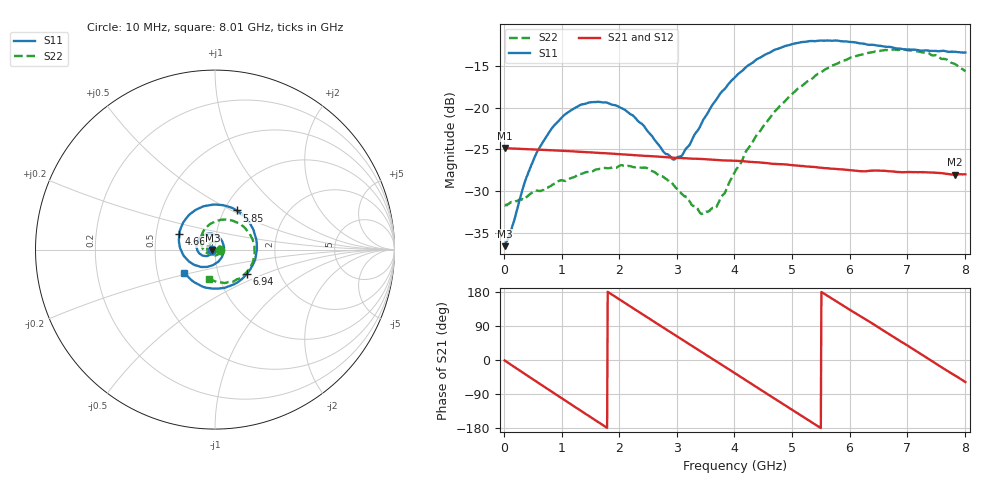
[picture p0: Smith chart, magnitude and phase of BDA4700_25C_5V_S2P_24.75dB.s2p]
!Agilent Technologies,E5071B,MY42404982,A.09.10
!Date: Mon Oct 20 13:38:55 2025
!Data & Calibration Information:
!Freq	S11:SOLT2(ON)	S21:SOLT2(ON)	S12:SOLT2(ON)	S22:SOLT2(ON)
# Hz S RI R 50
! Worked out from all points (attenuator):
!   801 points, 10 MHz to 8.01 GHz, reference 50 ohm
!   highest |S21| = -24.83 dB at 20 MHz (marker M1); lowest = -28.0 dB at 7.83 GHz (marker M2)
!   lowest |S11| = -36.6 dB at 10 MHz (marker M3), VSWR 1.03, Z = 48.5 - j0.135 ohm
!   |S11| at or under -10 dB: start of sweep to end of sweep
!   |S22| runs from -32.7 to -13.1 dB; largest |S21 - S12| = 0.00043
!   S11 on the Smith chart (normalised r, x): 10 MHz: 0.97, -0.00; 4.66 GHz: 0.66, +0.12; 5.85 GHz: 1.14, +0.53; 6.94 GHz: 1.37, -0.39; 8.01 GHz: 0.69, -0.19
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1e7  -0.0148 -0.00139  0.0573 -0.00126  0.0574 -0.0013  0.0261 -0.000838
2e7  -0.0152 -0.00212  0.0573 -0.00212  0.0573 -0.00237  0.026 -0.00106
3.8e8  -0.0263 -0.0267  0.0441 -0.0353  0.0441 -0.0353  0.0214 -0.0196
5.9e8  -0.0428 -0.0357  0.0282 -0.0484  0.0282 -0.0485  0.0134 -0.029
1e9  -0.0837 -0.0238  -0.0102 -0.0542  -0.0103 -0.0543  -0.0146 -0.0338
1.35e9  -0.1034 0.0137  -0.0388 -0.0381  -0.0388 -0.0381  -0.0361 -0.0179
2.07e9  -0.0424 0.0885  -0.0469 0.0235  -0.047 0.0236  -0.0304 0.0332
2.68e9  0.0408 0.0441  -0.00337 0.0508  -0.00338 0.0508  0.0129 0.0374
2.92e9  0.0493 0.00288  0.0168 0.0473  0.0168 0.0473  0.0246 0.0253
3.05e9  0.0462 -0.0214  0.0265 0.0424  0.0264 0.0425  0.0272 0.0154
3.44e9  -0.00348 -0.082  0.0463 0.017  0.0463 0.017  0.0185 -0.0141
3.69e9  -0.0569 -0.0965  0.0485 -0.00337  0.0485 -0.00353  0.000435 -0.0255
4.01e9  -0.1316 -0.0751  0.0394 -0.0276  0.0394 -0.0276  -0.0323 -0.0257
4.66e9  -0.199 0.0878  -0.00672 -0.0456  -0.00665 -0.0457  -0.0795 0.045
5.35e9  -0.052 0.2438  -0.0428 -0.0114  -0.0428 -0.0115  -0.0153 0.1478
5.85e9  0.1199 0.2179  -0.0359 0.0232  -0.0359 0.0232  0.0961 0.1616
6.25e9  0.2149 0.1082  -0.0143 0.0391  -0.0139 0.0393  0.1797 0.1058
6.68e9  0.2244 -0.0506  0.0152 0.0388  0.0154 0.0389  0.2201 -0.000305
6.94e9  0.1772 -0.1349  0.0294 0.0287  0.0296 0.0285  0.2109 -0.0709
7.38e9  0.0356 -0.2152  0.041 0.00132  0.0411 0.00129  0.134 -0.1621
7.83e9  -0.1245 -0.1757  0.0301 -0.026  0.0302 -0.0261  0.0129 -0.1813
8.01e9  -0.1703 -0.1285  0.021 -0.0339  0.0211 -0.0339  -0.0307 -0.1615
